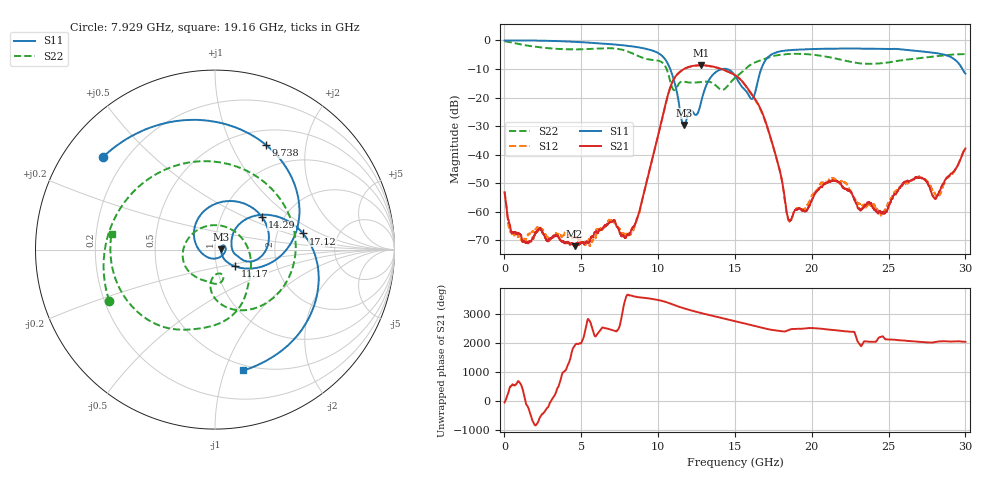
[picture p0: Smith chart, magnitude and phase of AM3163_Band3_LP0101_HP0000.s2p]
!Agilent Technologies,E8364B,MY43040894,A.07.50.67
!Agilent E8364B: A.07.50.67
!Date: Thursday, August 20, 2020 12:14:16
!Correction: S11(Full 2 Port(1,2))
!S21(Full 2 Port(1,2))
!S12(Full 2 Port(1,2))
!S22(Full 2 Port(1,2))
!S2P File: Measurements: S11, S21, S12, S22:
# Hz S  dB  R 50
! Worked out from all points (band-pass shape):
!   3201 points, 10 MHz to 30 GHz, reference 50 ohm
!   highest |S21| = -8.69 dB at 12.79 GHz (marker M1); lowest = -72.1 dB at 4.565 GHz (marker M2)
!   |S21| within 3 dB of the highest: 11.28 GHz to 14.85 GHz (3.575 GHz wide, 27.4 % of centre)
!   lowest |S11| = -29.6 dB at 11.68 GHz (marker M3), VSWR 1.07, Z = 53.4 + j0.17 ohm
!   |S11| at or under -10 dB: 10.79 GHz to 14.19 GHz (3.404 GHz wide, 27.3 % of centre); 14.47 GHz to 16.71 GHz (2.246 GHz wide, 14.4 % of centre); 29.8 GHz to end of sweep
!   |S22| runs from -17.4 to -0.3 dB; largest |S21 - S12| = 0.0053
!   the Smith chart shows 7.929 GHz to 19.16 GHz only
!   S11 on the Smith chart (normalised r, x): 7.929 GHz: 0.12, +0.36; 9.738 GHz: 0.68, +1.36; 11.17 GHz: 1.22, -0.23; 14.29 GHz: 1.56, +0.63; 17.12 GHz: 2.80, +0.67; 19.16 GHz: 0.45, -1.16
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1e7  -0.01 -1.9  -53.31 -44.4  -52.94 107.3  -0.26 -6.3
1.012791e9  -0.00 -27.7  -67.87 -97.3  -69.29 -177.6  -1.37 -83.3
2.249878e9  -0.07 -61.7  -65.99 97.6  -66.07 -173.2  -2.37 -162.8
4.564731e9  -0.48 -123.6  -72.10 104.5  -68.80 -73.8  -3.14 74.2
5.014581e9  -0.61 -135.6  -70.72 -141.2  -70.58 155.2  -3.09 49.6
6.917072e9  -1.30 171.9  -63.70 -56.5  -62.90 -65.7  -2.72 -71.1
7.929234e9  -1.83 140.4  -68.67 4.8  -68.07 -8.9  -3.68 -154.2
9.738006e9  -3.75 64.2  -39.12 -93.9  -39.18 -94.9  -6.87 14.2
1.000979e10  -4.43 47.6  -33.08 -120.8  -33.17 -121.7  -7.09 -16.8
1.11719e10  -16.84 -40.1  -12.34 43.6  -12.39 43.7  -16.86 -74.3
1.167798e10  -29.64 2.8  -10.03 -44.8  -10.11 -44.9  -14.43 -91.5
1.279324e10  -21.75 -171.7  -8.69 152.4  -8.75 152.5  -14.61 -125.4
1.429274e10  -9.93 34.6  -10.34 -35.9  -10.39 -35.4  -17.13 66.6
1.5005e10  -12.36 -13.2  -12.15 -124.6  -12.19 -124.5  -13.12 -24.9
1.612025e10  -20.51 12.1  -19.02 90.6  -19.24 90.7  -8.18 -78.8
1.712304e10  -6.05 10.4  -30.57 -39.0  -30.82 -36.5  -6.10 -116.2
1.847259e10  -3.44 -54.7  -62.56 -76.6  -62.82 -78.2  -4.75 -164.7
1.915674e10  -3.21 -76.8  -58.93 -28.2  -59.01 -29.5  -4.69 171.6
2.000958e10  -3.02 -100.0  -55.85 -4.0  -54.43 -7.9  -4.95 141.0
2.27368e10  -2.83 -162.7  -55.19 -133.7  -54.92 -126.3  -7.71 19.7
2.500479e10  -3.00 144.3  -58.34 -38.0  -57.03 -39.0  -7.70 -92.9
3e10  -11.62 -28.5  -37.85 -119.3  -37.62 -115.5  -4.78 101.2
